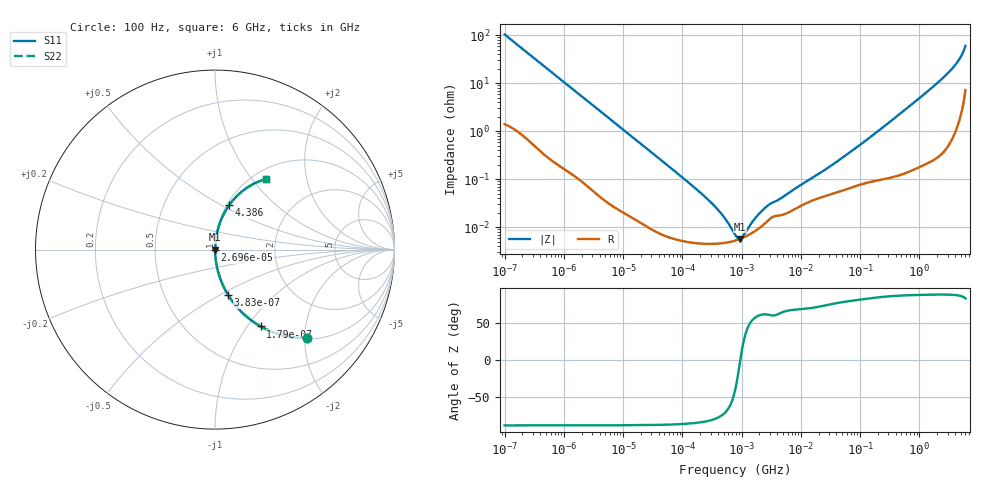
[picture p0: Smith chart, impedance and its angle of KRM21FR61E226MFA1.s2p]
!Murata Part Number: KRM21FR61E226MFA1
!These Parameters are Measured in Series Mode Connection
!Data Generated on Jan 08, 2026
!  o--ll--o
!Port1  Port2
!  o------o
!Operation Temp=25[degC], DC Bias Voltage=0[V]
!Freq. Start=100[Hz] Stop=6[GHz] 401[Steps]
# Hz S RI R 50
!Freq.(Hz) S11(Real) S11(Imag) S21(Real) S21(Imag) S12(Real) S12(Imag) S22(Real) S22(Imag)
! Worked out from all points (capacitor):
!   401 points, 100 Hz to 6 GHz, reference 50 ohm
!   read as one part in series: C = 15.4 uF near 109 Hz
!   lowest |Z| = 5.71 mohm at 926.5 kHz (marker M1)
!   series resonance near 953.7 kHz, so ESL is about 1.8 nH
!   S11 on the Smith chart (normalised r, x): 100 Hz: 1.03, -2.06; 179 Hz: 1.02, -1.16; 383 Hz: 1.01, -0.55; 26.96 kHz: 1.00, -0.01; 4.386 GHz: 1.02, +0.54; 6 GHz: 1.14, +1.18
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100  0.5144 -0.4931  0.4856 0.4931  0.4856 0.4931  0.5144 -0.4931
179  0.2549 -0.428  0.7451 0.428  0.7451 0.428  0.2549 -0.428
383  0.0726 -0.2522  0.9274 0.2522  0.9274 0.2522  0.0726 -0.2522
820  0.018 -0.1258  0.982 0.1258  0.982 0.1258  0.018 -0.1258
2008  0.00367 -0.0527  0.9963 0.0527  0.9963 0.0527  0.00367 -0.0527
26957  0.000114 -0.00404  0.9999 0.00404  0.9999 0.00404  0.000114 -0.00404
40335  8.21e-05 -0.00271  0.9999 0.00271  0.9999 0.00271  8.21e-05 -0.00271
231233  4.55e-05 -0.000449  1 0.000449  1 0.000449  4.55e-05 -0.000449
395726  4.56e-05 -0.00023  1 0.00023  1 0.00023  4.56e-05 -0.00023
647581  4.97e-05 -9.05e-05  1 9.05e-05  1 9.05e-05  4.97e-05 -9.05e-05
774597  5.26e-05 -4.74e-05  0.9999 4.74e-05  0.9999 4.74e-05  5.26e-05 -4.74e-05
926525  5.67e-05 -6.4e-06  0.9999 6.4e-06  0.9999 6.4e-06  5.67e-05 -6.4e-06
1325623  6.95e-05 7.34e-05  0.9999 -7.34e-05  0.9999 -7.34e-05  6.95e-05 7.34e-05
1983483  9.57e-05 0.000167  0.9999 -0.000167  0.9999 -0.000167  9.57e-05 0.000167
2837864  0.00014 0.000253  0.9999 -0.000253  0.9999 -0.000253  0.00014 0.000253
1.555665e7  0.000359 0.001  0.9996 -0.001  0.9996 -0.001  0.000359 0.001
5.211241e7  0.000594 0.00283  0.9994 -0.00283  0.9994 -0.00283  0.000594 0.00283
3.124326e8  0.00129 0.0153  0.9987 -0.0153  0.9987 -0.0153  0.00129 0.0153
1.712697e9  0.00948 0.0834  0.9905 -0.0834  0.9905 -0.0834  0.00948 0.0834
2.931063e9  0.0275 0.1495  0.9725 -0.1495  0.9725 -0.1495  0.0275 0.1495
4.385646e9  0.0789 0.2478  0.9211 -0.2478  0.9211 -0.2478  0.0789 0.2478
6e9  0.2845 0.3948  0.7155 -0.3948  0.7155 -0.3948  0.2845 0.3948
